TYPE ST_ControlOutput_UINT_TO_BIT :
STRUCT
	Set_digital_output				:	BIT;
	Enable_thresholds_output		:	BIT;
	Set_tristate					:	BIT;
	Disalbe_thresholds_cw			:	BIT;
	Disalbe_thresholds_ccw			:	BIT;
	{attribute 'hide'}
	reserve_b6						:	BIT;
	{attribute 'hide'}
	reserve_b7						:	BIT;
	{attribute 'hide'}
	reserve_b8						:	BIT;
	{attribute 'hide'}
	reserve_byte					:	BIT;
	
END_STRUCT
END_TYPE
